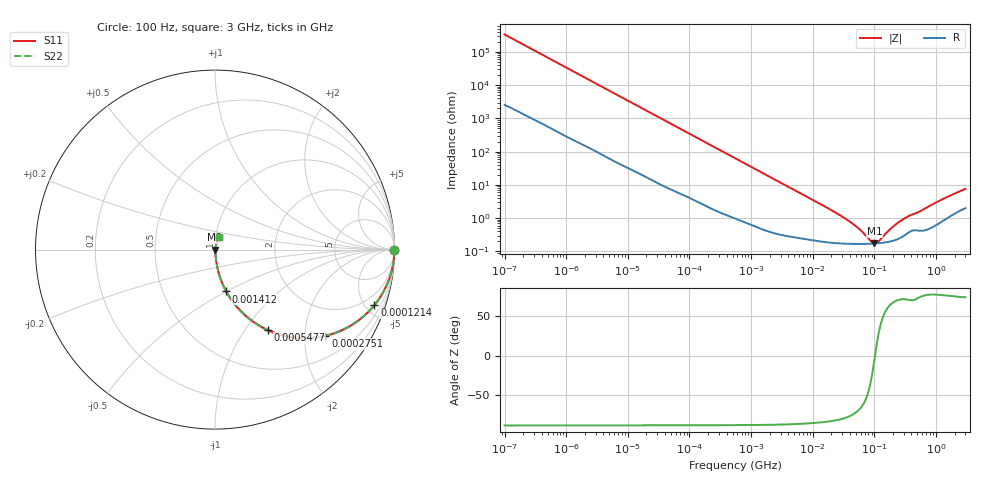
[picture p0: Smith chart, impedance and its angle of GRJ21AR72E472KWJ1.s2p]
!Murata Part Number: GRJ21AR72E472KWJ1
!These Parameters are Measured in Series Mode Connection
!Data Generated on Jun 19, 2026
!  o--ll--o
!Port1  Port2
!  o------o
!Operation Temp=25[degC], DC Bias Voltage=0[V]
!Freq. Start=100[Hz] Stop=3[GHz] 401[Steps]
# Hz S RI R 50
!Freq.(Hz) S11(Real) S11(Imag) S21(Real) S21(Imag) S12(Real) S12(Imag) S22(Real) S22(Imag)
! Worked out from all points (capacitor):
!   401 points, 100 Hz to 3 GHz, reference 50 ohm
!   read as one part in series: C = 4.78 nF near 109 Hz
!   lowest |Z| = 175 mohm at 100.1 MHz (marker M1)
!   series resonance near 102.6 MHz, so ESL is about 500 pH
!   S11 on the Smith chart (normalised r, x): 100 Hz: open; 121.4 kHz: 1.07, -5.71; 275.1 kHz: 1.03, -2.53; 547.7 kHz: 1.02, -1.28; 1.412 MHz: 1.01, -0.50; 3 GHz: 1.04, +0.15
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100  1 -0.000301  2.4e-06 0.000301  2.4e-06 0.000301  1 -0.000301
1788  0.9999 -0.0053  7.48e-05 0.0053  7.48e-05 0.0053  0.9999 -0.0053
10443  0.9988 -0.0306  0.00123 0.0306  0.00123 0.0306  0.9988 -0.0306
31977  0.9905 -0.0921  0.0095 0.0921  0.0095 0.0921  0.9905 -0.0921
69391  0.9592 -0.1924  0.0408 0.1924  0.0408 0.1924  0.9592 -0.1924
121426  0.8878 -0.3097  0.1122 0.3097  0.1122 0.3097  0.8878 -0.3097
178874  0.7877 -0.4028  0.2123 0.4028  0.2123 0.4028  0.7877 -0.4028
275091  0.6148 -0.4802  0.3852 0.4802  0.3852 0.4802  0.6148 -0.4802
547723  0.2933 -0.4476  0.7067 0.4476  0.7067 0.4476  0.2933 -0.4476
842342  0.1528 -0.3513  0.8472 0.3513  0.8472 0.3513  0.1528 -0.3513
1411895  0.063 -0.2334  0.937 0.2334  0.937 0.2334  0.063 -0.2334
3339322  0.0141 -0.1046  0.9859 0.1046  0.9859 0.1046  0.0141 -0.1046
9794414  0.00349 -0.0362  0.9965 0.0362  0.9965 0.0362  0.00349 -0.0362
4.0536e7  0.00175 -0.00755  0.9982 0.00755  0.9982 0.00755  0.00175 -0.00755
5.9714e7  0.0017 -0.00402  0.9983 0.00402  0.9983 0.00402  0.0017 -0.00402
8.79653e7  0.00172 -0.00109  0.9983 0.00109  0.9983 0.00109  0.00172 -0.00109
1.000898e8  0.00174 -0.000174  0.9983 0.000174  0.9983 0.000174  0.00174 -0.000174
1.188943e8  0.00178 0.00105  0.9982 -0.00105  0.9982 -0.00105  0.00178 0.00105
1.751444e8  0.00198 0.00399  0.998 -0.00399  0.998 -0.00399  0.00198 0.00399
3.340322e8  0.00347 0.0102  0.9965 -0.0102  0.9965 -0.0102  0.00347 0.0102
1.443257e9  0.0109 0.0397  0.9891 -0.0397  0.9891 -0.0397  0.0109 0.0397
3e9  0.0247 0.07  0.9753 -0.07  0.9753 -0.07  0.0247 0.07
